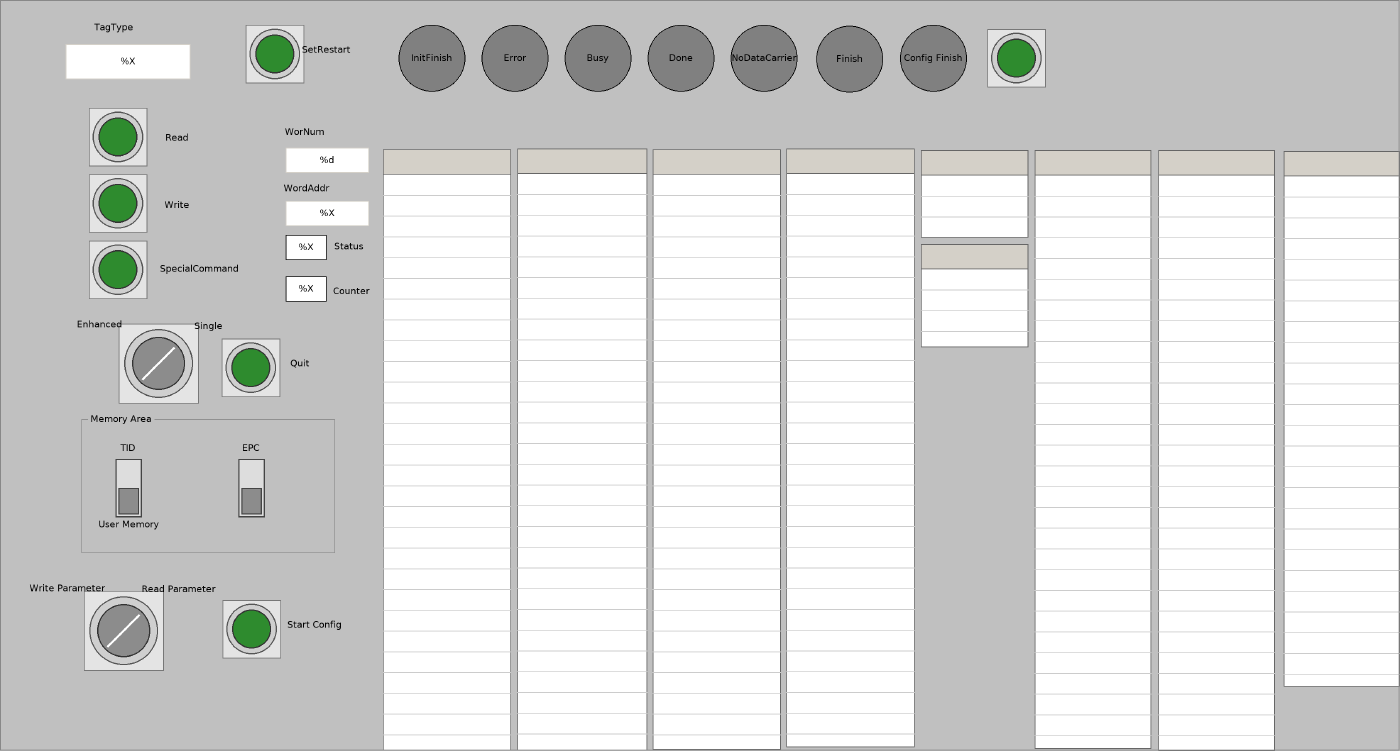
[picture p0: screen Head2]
VISUALIZATION Head2  // 1686x905
    GroupBox (98,497 305x169), "Memory Area"
        DipSwitch (22,56 70x70), variable: MAIN.Head2UserMemoryUID, behaviour: TOGGLE, style: Switch-DipSwitch-Gray
        DipSwitch (170,56 70x70), variable: MAIN.Head2EPC, behaviour: TOGGLE, style: Switch-DipSwitch-Gray
        Label (129,28 150x30), "EPC"
    PushSwitch (107,130 70x70), variable: MAIN.Head2Read, behaviour: TAP, style: Switch-PushSwitch-Green
    PushSwitch (107,210 70x70), variable: MAIN.Head2Write, behaviour: TAP, style: Switch-PushSwitch-Green
    RotarySwitch (138,390 106x96), variable: MAIN.Head2SingleEnhanced, behaviour: TOGGLE, style: Switch-RotarySwitch-Gray
    Textfield (79,53 150x42), "%X", tooltip "TagType", text variable: MAIN.Head2TagType
        OnMouseDown: write MAIN.Head1TagType via Default
    Table (461,180 154x724), data array: MAIN.IC_KP2_2HB21_IUH_MF_Head2.IDENTControl_FB_MF.INDATA
        p1892666644: MAIN.Data_Channel.InData[2][INDEX]
        p3854506369: MAIN.IC_KP2_2HB21_IUH_MF_Head2.IDENTControl_FB_MF.INDATA[INDEX]
    Table (623,179 156x725), data array: MAIN.IC_KP2_2HB21_IUH_MF_Head2.IDENTControl_FB_MF.OUTDATA
        p1892666644: MAIN.Data_Channel.OutData[2][INDEX]
        p3854506369: MAIN.IC_KP2_2HB21_IUH_MF_Head2.IDENTControl_FB_MF.OUTDATA[INDEX]
        Columns.Column.[0].Template: OnMouseDown: write the text variable via Default
    Textfield (344,242 100x30), "%X", text variable: MAIN.Head2StartAddress
        OnMouseClick: write MAIN.Head1StartAddress via Default
    Textfield (344,178 100x30), "%d", text variable: MAIN.Head2WordNum
        OnMouseClick: write MAIN.Head1WordNum via Default
    PushSwitch (296,30 70x70), variable: MAIN.Head2SetRestart, behaviour: TAP, style: Switch-PushSwitch-Green
    PushSwitch (267,408 70x70), tooltip "Cancel "Enhanced"-Command", variable: MAIN.Head2Quit, behaviour: TAP, style: Switch-PushSwitch-Green
    PushSwitch (107,290 70x70), variable: MAIN.Head2SpecialCommand, behaviour: TAP, style: Switch-PushSwitch-Green
    Table (1546,182 140x645), data array: MAIN.Head2Data.SpecialCommand
        p1892666644: MAIN.Data_Channel.SpecialCommand[2][INDEX]
        p3854506369: MAIN.Head2Data.SpecialCommand[INDEX]
        Columns.Column.[0].Template: OnMouseDown: write the text variable via Default
    Rectangle (344,283 49x30), "%X", text variable: MAIN.Head2Status, input disabled if: TRUE
    Rectangle (344,333 49x30), "%X", text variable: MAIN.Head2ReplyCounter, input disabled if: TRUE
    Ellipse (480,30 80x80), "InitFinish", colour toggle: MAIN.Head2InitFinish
    Ellipse (580,30 80x80), "Error", colour toggle: MAIN.Head2Error
    Ellipse (680,30 80x80), "Busy", colour toggle: MAIN.Head2Busy
    Ellipse (780,30 80x80), "Done", colour toggle: MAIN.Head2Done
    Ellipse (880,30 80x80), "NoDataCarrier", colour toggle: MAIN.Head2NoDataCarrier
    Label (62,18 150x30), "TagType"
    Label (292,144 150x30), "WorNum"
    Label (294,212 150x30), "WordAddr"
    Label (347,283 146x28), "Status"
    Label (346,336 154x30), "Counter"
    Label (138,151 150x30), "Read"
    Label (138,232 150x30), "Write"
    Label (165,309 150x30), "SpecialCommand"
    Label (45,376 150x30), "Enhanced"
    Label (176,378 150x30), "Single"
    Label (286,423 150x30), "Quit"
    Label (79,525 150x30), "TID"
    Label (80,617 150x30), "User Memory"
    Ellipse (983,31 80x80), "Finish", colour toggle: MAIN.Head2Finish
    Table (786,180 154x723), data array: MAIN.Head2Data.ReadData
        p1892666644: MAIN.Data_Channel.SpecialCommand[2][INDEX]
        p3854506369: MAIN.Head2Data.ReadData[INDEX]
        Columns.Column.[0].Template: OnMouseDown: write the text variable via Default
    Table (947,179 154x721), data array: MAIN.Head2Data.ReadData
        p1892666644: MAIN.Data_Channel.SpecialCommand[2][INDEX]
        p3854506369: MAIN.Head2Data.ReadData[INDEX]
        p2232123230: WriteData
        Columns.Column.[0].Template: OnMouseDown: write the text variable via Default
    Label (318,45 150x30), "SetRestart"
    RotarySwitch (96,712 106x96), variable: MAIN.Head2WriteParameter, behaviour: TOGGLE, style: Switch-RotarySwitch-Gray
    Label (140,695 150x30), "Read Parameter"
    Label (6,694 150x30), "Write Parameter"
    PushSwitch (268,723 70x70), variable: MAIN.Head2StartConfig, behaviour: TAP, style: Switch-PushSwitch-Green
    Label (304,739 150x28), "Start Config"
    Ellipse (1084,30 80x80), "Config Finish", colour toggle: MAIN.Head2EndConfig
    PushSwitch (1189,35 70x70), variable: MAIN.Head2NewData, behaviour: TAP, style: Switch-PushSwitch-Green
    Table (1109,181 129x105), data array: MAIN.Head2Data.NumberTags
        p1892666644: MAIN.Data_Channel.SpecialCommand[2][INDEX]
        p3854506369: MAIN.Head2Data.NumberTags[INDEX]
        Columns.Column.[0].Template: OnMouseDown: write the text variable via Default
    Table (1246,181 140x721), data array: MAIN.Head2Data.EPC_LeaveTag
        p1892666644: MAIN.Data_Channel.SpecialCommand[2][INDEX]
        p3854506369: MAIN.Head2Data.EPC_LeaveTag[INDEX]
        Columns.Column.[0].Template: OnMouseDown: write the text variable via Default
    Table (1395,181 140x724), data array: MAIN.Head2Data.EPC_WrittenTag
        p1892666644: MAIN.Data_Channel.SpecialCommand[2][INDEX]
        p3854506369: MAIN.Head2Data.EPC_WrittenTag[INDEX]
        Columns.Column.[0].Template: OnMouseDown: write the text variable via Default
    Table (1109,294 129x124), data array: MAIN.Head2Data.TagInformation
        p1892666644: MAIN.Data_Channel.SpecialCommand[2][INDEX]
        p3854506369: MAIN.Head2Data.TagInformation[INDEX]
        Columns.Column.[0].Template: OnMouseDown: write the text variable via Default
END_VISUALIZATION
